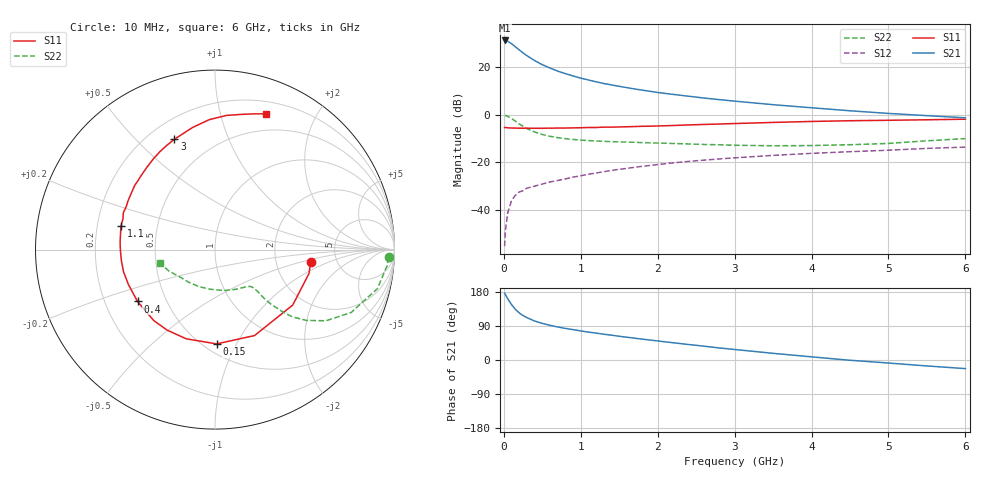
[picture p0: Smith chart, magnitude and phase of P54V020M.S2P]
! SIEMENS Small Signal Semiconductors
! BFP183
! Si NPN RF Bipolar Junction Transistor in SOT143
! VCE = 4 V  IC = 20 mA
! Common Emitter S-Parameters:  March  1996
# GHz  S  MA  R  50
!  f  S11  S21  S12  S22
! GHz  MAG  ANG  MAG  ANG  MAG  ANG  MAG  ANG
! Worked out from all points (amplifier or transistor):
!   36 points, 10 MHz to 6 GHz, reference 50 ohm
!   highest |S21| = 31.4 dB at 10 MHz (marker M1)
!   |S21| within 3 dB of that: start of sweep to 162.9 MHz
!   unconditionally stable (mu >= 1): 839.9 MHz to 5.603 GHz
!   at 250 MHz: K = 0.48, MSG = 29.0 dB, |S12| = -32.0 dB
!   at 1.4 GHz: K = 1.12, MAG = 15.9 dB, |S12| = -23.4 dB
!   at 6 GHz: K = 0.96, MSG = 6.2 dB, |S12| = -13.6 dB
!   S11 on the Smith chart (normalised r, x): 10 MHz: 3.20, -0.60; 150 MHz: 0.58, -0.84; 400 MHz: 0.34, -0.27; 1.1 GHz: 0.30, +0.11; 3 GHz: 0.30, +0.65; 6 GHz: 0.32, +1.40
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0.01  0.5379 -7.1  36.99 176.1  0.0017 89.0  0.9695 -2.6
0.02  0.5404 -14.3  36.83 172.8  0.0036 78.2  0.9624 -5.5
0.05  0.532 -35.5  35.58 161.6  0.0085 80.0  0.9307 -13.5
0.1  0.5272 -65.3  31.5 146.1  0.0156 65.5  0.8358 -24.8
0.15  0.5254 -89.0  27.21 133.7  0.0201 58.3  0.7342 -32.7
0.2  0.5223 -107.8  23.43 124.3  0.0236 53.4  0.6435 -37.8
0.25  0.5219 -120.6  20.19 117.1  0.0252 50.8  0.5708 -41.0
0.3  0.5223 -130.7  17.68 111.8  0.0284 50.0  0.5131 -42.6
0.4  0.5195 -146.2  13.95 102.8  0.0313 48.8  0.4344 -44.3
0.5  0.5201 -158.1  11.4 96.6  0.0347 49.0  0.3844 -44.8
0.6  0.5243 -166.3  9.711 91.5  0.0384 50.0  0.3519 -44.6
0.7  0.5252 -173.3  8.338 87.2  0.0413 50.8  0.3298 -44.5
0.9  0.5303 175.6  6.603 80.2  0.0486 52.2  0.3026 -44.9
1.1  0.5401 165.9  5.428 73.6  0.0559 52.8  0.2857 -46.0
1.5  0.5549 151.2  3.987 62.6  0.0708 52.3  0.2688 -50.3
1.8  0.573 141.1  3.315 55.0  0.0822 51.2  0.2591 -55.3
2.2  0.5952 129.6  2.695 45.5  0.0969 48.4  0.2485 -62.9
3  0.6552 110.2  1.943 27.7  0.1239 41.8  0.2279 -82.8
3.5  0.6914 100.5  1.636 17.6  0.1395 37.5  0.2226 -97.5
4.5  0.7507 85.0  1.217 -0.7  0.1668 28.5  0.2342 -129.8
5.5  0.7863 74.1  0.961 -15.7  0.196 20.9  0.2831 -155.0
6  0.8082 69.3  0.865 -22.7  0.2085 16.3  0.3157 -165.9
